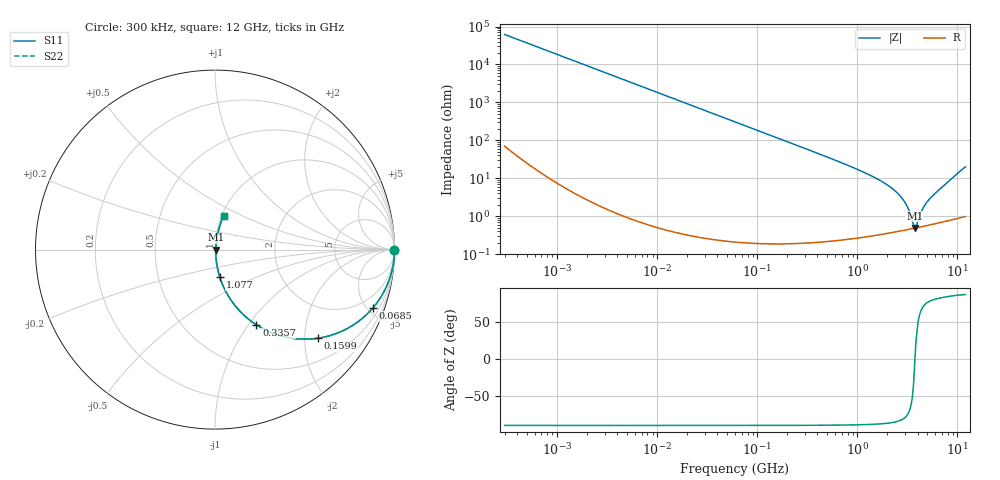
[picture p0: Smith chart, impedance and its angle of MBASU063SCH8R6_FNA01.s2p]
! MBASU063SCH8R6_FNA01  S-PARAMETER MODEL  ( General Type )
! Model Generated by TAIYO YUDEN Corporation (http://www.ty-top.com)
! Version 1.0
! TAIYO YUDEN Control No. 130801
! Copyright(c) 2013 TAIYO YUDEN CO.,LTD. All Rights Reserved.
! Product Description (link to TY-COMPAS)
! https://ds.yuden.co.jp/TYCOMPAS/or/detail?pn=MBASU063SCH8R6DFNA01&u=M
! Products Name : Multilayer Ceramic Capacitors
! Characteristics :
!  Capacitance : 8.6 pF , Rated Voltage : 50V , TCC : CH / C0H
!  Case Size : 0.6 x 0.3 / 0.024 x 0.012 [mm/inch] , Thickness : 0.3 / 0.012 [mm/inch]
!  (Conditions: Temperature = 25 degC , DC Bias Current/Voltage = 0A / 0V)
! External Node Assignments :
!  1  o---| |---o  2
! GND o---------o GND
! Frequency Range : 0.3MHz  -  12000MHz  [ 401 STEP ]
# MHz S RI R 50
! Freq[MHz].  S11 Real  S11 Imag  S21 Real  S21 Imag  S12 Real  S12 Imag  S22 Real  S22 Imag
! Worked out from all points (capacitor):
!   401 points, 300 kHz to 12 GHz, reference 50 ohm
!   read as one part in series: C = 8.6 pF near 316.3 kHz
!   lowest |Z| = 489 mohm at 3.741 GHz (marker M1)
!   series resonance near 3.761 GHz, so ESL is about 210 pH
!   S11 on the Smith chart (normalised r, x): 300 kHz: open; 68.5 MHz: 1.00, -5.40; 159.9 MHz: 1.00, -2.31; 335.7 MHz: 1.00, -1.09; 1.077 GHz: 1.01, -0.32; 12 GHz: 1.02, +0.40
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0.3  1 -0.00162  4.47e-06 0.00162  4.47e-06 0.00162  1 -0.00162
1.769972  0.9999 -0.00956  9.44e-05 0.00956  9.44e-05 0.00956  0.9999 -0.00956
10.44266  0.9968 -0.0562  0.00319 0.0562  0.00319 0.0562  0.9968 -0.0562
26.39317  0.98 -0.1398  0.02 0.1398  0.02 0.1398  0.98 -0.1398
60  0.9047 -0.2933  0.0953 0.2933  0.0953 0.2933  0.9047 -0.2933
68.49786  0.8792 -0.3255  0.1208 0.3255  0.1208 0.3255  0.8792 -0.3255
101.9188  0.7668 -0.4224  0.2332 0.4224  0.2332 0.4224  0.7668 -0.4224
159.8975  0.5715 -0.494  0.4285 0.494  0.4285 0.494  0.5715 -0.494
335.7268  0.231 -0.4197  0.769 0.4197  0.769 0.4197  0.231 -0.4197
353.9943  0.2126 -0.4072  0.7874 0.4072  0.7874 0.4072  0.2126 -0.4072
585.5907  0.0885 -0.2804  0.9115 0.2804  0.9115 0.2804  0.0885 -0.2804
1076.992  0.0268 -0.1531  0.9732 0.1531  0.9732 0.1531  0.0268 -0.1531
2088.533  0.00731 -0.0607  0.9927 0.0607  0.9927 0.0607  0.00731 -0.0607
2514.07  0.00558 -0.0404  0.9944 0.0404  0.9944 0.0404  0.00558 -0.0404
2947.191  0.00485 -0.0241  0.9952 0.0241  0.9952 0.0241  0.00485 -0.0241
3190.978  0.00471 -0.0162  0.9953 0.0162  0.9953 0.0162  0.00471 -0.0162
3547.679  0.00474 -0.0058  0.9953 0.0058  0.9953 0.0058  0.00474 -0.0058
3740.715  0.00484 -0.000473  0.9952 0.000473  0.9952 0.000473  0.00484 -0.000473
3944.255  0.005 0.00382  0.995 -0.00382  0.995 -0.00382  0.005 0.00382
4623.766  0.00573 0.0169  0.9943 -0.0169  0.9943 -0.0169  0.00573 0.0169
5278.635  0.00666 0.028  0.9933 -0.028  0.9933 -0.028  0.00666 0.028
12000  0.0475 0.1896  0.9525 -0.1896  0.9525 -0.1896  0.0475 0.1896
